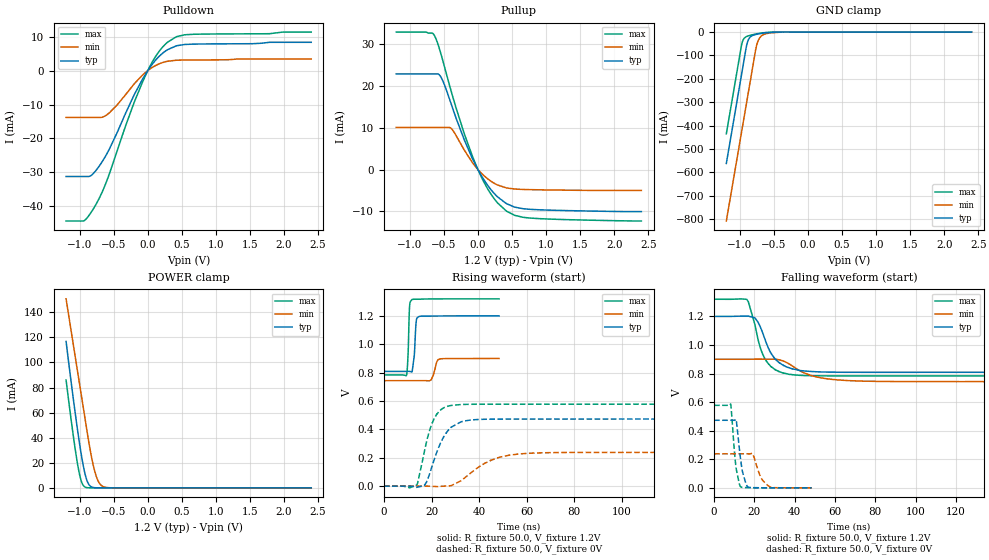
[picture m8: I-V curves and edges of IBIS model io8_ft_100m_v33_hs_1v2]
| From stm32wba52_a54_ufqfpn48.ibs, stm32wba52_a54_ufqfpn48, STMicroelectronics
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[Model]   io8_ft_100m_v33_hs_1v2
Model_type I/O
Polarity   Non-Inverting
Enable   Active-Low
| CAP_THRESHOLD on pad IOFT is "UDTCAPC" :
| Rising=30.0% of vddiom   Falling=70.0% of vddiom
| C_comp min and max val. don't necessarily correlate with the min and max pvt
| but are the smallest and greatest pad capacitance found.
| var   typ   min   max
C_comp   1.83455pF  1.64924pF  1.97633pF
|C_comp_pullup   1.12540pF  1.02622pF  1.16140pF
|C_comp_pulldown   709.14500fF  623.02001fF  814.93000fF
Vinl = 450.0mV
Vinh = 660.0mV
Vmeas = 600.0mV   | Reference voltage for timing measurements
Cref  = 50.0pF   | Timing specification test load capacitance value
Rref  = 1.0MOhm   | Timing specification test load resistance value
Vref  = 660.0mV   | Timing specification test load voltage
[Model Spec]
| TIME_THRESHOLD on pin ZIV33M is "CMOS" :
| Rising=50.0% of vddiom   Falling=50.0% of vddiom
Vinl 436.50000mV 342.50000mV 466.50000mV
Vinh 753.50000mV 549.50000mV 839.50000mV
| variable   typ   min   max
[Temperature Range] 25.0 140.0 -40.0
| variable   typ   min   max
[Voltage Range] 1.2V 900.0mV 1.32V
| variable   typ   min   max
[POWER Clamp Reference] 1.2V 900.0mV 1.32V
| variable   typ   min   max
[GND Clamp Reference] 0V 0V 0V
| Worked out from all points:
|   slope of the pulldown table from 0 to 0.18 V, typ, clamps not added: 40.6 ohm
|   slope of the pullup table from 0 to 0.18 V, typ, clamps not added: 39.4 ohm
|   GND clamp passes 1 mA (typ) near -0.51 V on its own axis
|   POWER clamp passes 1 mA (typ) near -0.83 V on its own axis
|   rising waveform, R_fixture 50.0, V_fixture 1.2V: 20-80 % time 880ps typ, 1.54ns min, 594ps max; typ from 0.809 V to 1.2 V
|   falling waveform, R_fixture 50.0, V_fixture 1.2V: 20-80 % time 8.36ns typ, 14.3ns min, 6.93ns max; typ from 1.2 V to 0.809 V
|   rising waveform, R_fixture 50.0, V_fixture 0V: 20-80 % time 7.01ns typ, 13.1ns min, 5.38ns max; typ from 0 V to 0.473 V
|   falling waveform, R_fixture 50.0, V_fixture 0V: 20-80 % time 2.69ns typ, 4.09ns min, 2.23ns max; typ from 0.473 V to 0 V
[POWER Clamp]
-1.2V     116.7mA    150.7mA    85.92mA
-1.06V    57.23mA    102.6mA    28.68mA
-1.02V    41.75mA    88.91mA    15.5mA
-980mV    27.6mA     75.18mA    5.935mA
-920mV    10.75mA    54.6mA     597.6uA
-870mV    3.065mA    37.68mA    60.82uA
-820mV    594.6uA    22.85mA    5.912uA
-770mV    99.71uA    11.47mA    572nA
-730mV    23.34uA    5.552mA    88.29nA
-680mV    3.779uA    1.833mA    8.565nA
-510mV    7.889nA    23.13uA    53.67pA
2.4V      0A         0A         0A
[GND Clamp]
-1.2V     -561.6mA   -807.5mA   -434.8mA
-980mV    -187.6mA   -433.5mA   -60.76mA
-960mV    -153.6mA   -399.5mA   -38.21mA
-900mV    -54.17mA   -297.5mA   -18.87mA
-870mV    -29.55mA   -246.5mA   -15.73mA
-830mV    -17.05mA   -178.5mA   -12.57mA
-760mV    -9.921mA   -62.77mA   -8.045mA
-730mV    -8.191mA   -35.56mA   -6.403mA
-680mV    -5.826mA   -15.57mA   -4.089mA
-580mV    -2.43mA    -5.043mA   -1.157mA
-330mV    -11.72uA   -245.5uA   -300.5nA
2.4V      872pA      1.055uA    338.3pA
| variable   typ   min   max
[Pullup Reference] 1.2V 900.0mV 1.32V
| variable   typ   min   max
[Pulldown Reference] 0V 0V 0V
[Pullup]
-1.2V     22.83mA    10.05mA    32.83mA
-760mV    22.83mA    10.05mA    32.83mA
-640mV    22.82mA    10.05mA    32.02mA
-580mV    22.78mA    10.05mA    29.58mA
-540mV    21.98mA    10.05mA    27.42mA
-390mV    15.52mA    9.759mA    18.55mA
-200mV    7.069mA    4.63mA     8.528mA
-30mV     926.7uA    571.2uA    1.132mA
190mV     -4.777mA   -2.782mA   -5.837mA
420mV     -8.158mA   -4.403mA   -9.943mA
790mV     -9.528mA   -4.812mA   -11.62mA
2.4V      -10.04mA   -4.994mA   -12.3mA
[Pulldown]
-1.2V     -31.2mA    -13.81mA   -44.3mA
-940mV    -31.2mA    -13.81mA   -44.26mA
-850mV    -31.11mA   -13.81mA   -42.26mA
-760mV    -29.39mA   -13.81mA   -39.38mA
-660mV    -26.52mA   -13.68mA   -35.32mA
-560mV    -22.95mA   -12.35mA   -30.17mA
-330mV    -12.74mA   -7.204mA   -16.5mA
-80mV     -2.622mA   -1.37mA    -3.49mA
110mV     2.963mA    1.428mA    3.999mA
290mV     6.144mA    2.737mA    8.347mA
540mV     7.674mA    3.096mA    10.53mA
2.4V      8.319mA    3.393mA    11.34mA
[Ramp]
dV/dt_r 283.7949mV/6.92861ns 142.77217mV/13.00747ns 346.61957mV/5.26294ns
dV/dt_f 234.65831mV/8.27658ns 93.77058mV/13.83346ns 321.77305mV/6.57582ns
R_load = 50.0
| Removed startup time: 0s 0s 0s  .
| Removed end time: 48.4ns.
[Rising Waveform]
R_fixture   = 50.0
V_fixture   = 1.2V
V_fixture_min = 900.0mV
V_fixture_max = 1.32V
0s        808.9mV    743.7mV    783.7mV
9.5ns     808.9mV    743.7mV    782.2mV
10.15ns   809mV      743.7mV    932.1mV
10.8ns    808.5mV    743.7mV    1.272V
11.7ns    804.5mV    743.7mV    1.314V
12.75ns   918.6mV    743.7mV    1.318V
13.6ns    1.165V     743.7mV    1.317V
14.85ns   1.197V     743.7mV    1.317V
23.75ns   1.199V     897.3mV    1.32V
48.4ns    1.2V       899.8mV    1.32V
| Removed startup time: 0s 0s 0s  .
| Removed end time: 198.4ns.
[Falling Waveform]
R_fixture   = 50.0
V_fixture   = 1.2V
V_fixture_min = 900.0mV
V_fixture_max = 1.32V
0s        1.2V       900mV      1.32V
16.2ns    1.202V     900mV      1.32V
20.25ns   1.19V      900.9mV    1.143V
22.8ns    1.131V     901mV      986.3mV
24.95ns   1.052V     900.6mV    910.1mV
29.65ns   912.7mV    900.7mV    833.9mV
37.35ns   839.7mV    866.5mV    794.1mV
48.6ns    814.2mV    784.1mV    784.7mV
66.9ns    809mV      750.4mV    783.6mV
198.4ns   808.9mV    743.7mV    783.7mV
| Removed startup time: 0s 0s 0s  .
| Removed end time: 198.4ns.
[Rising Waveform]
R_fixture   = 50.0
V_fixture   = 0V
V_fixture_min = 0V
V_fixture_max = 0V
0s        4.839nV    985.4nV    4.249nV
13.75ns   -8.794mV   2.874uV    6.54mV
17.15ns   8.066mV    14.14uV    255.9mV
20.35ns   146.8mV    -1.516mV   448.2mV
24ns      312.2mV    -1.26mV    539.4mV
28.15ns   414.1mV    3.473mV    568.6mV
33.85ns   459.4mV    56.82mV    576.2mV
44.8ns    472.1mV    181.5mV    577.5mV
56.7ns    472.8mV    226.7mV    577.6mV
198.4ns   473mV      238mV      577.7mV
| Removed startup time: 0s 0s 0s  .
| Removed end time: 48.4ns.
[Falling Waveform]
R_fixture   = 50.0
V_fixture   = 0V
V_fixture_min = 0V
V_fixture_max = 0V
0s        473mV      238mV      577.7mV
8.25ns    473mV      238mV      585.4mV
10.95ns   476.8mV    238mV      137.2mV
13.05ns   211.5mV    238mV      9.113mV
14ns      118.7mV    238mV      2.926mV
16.95ns   4.445mV    238mV      1.571mV
18.9ns    1.6mV      241.8mV    850.7uV
23.7ns    581.6uV    60.1mV     261uV
27.35ns   291.5uV    9.579mV    129.5uV
48.4ns    10.51uV    152.8uV    503nV
